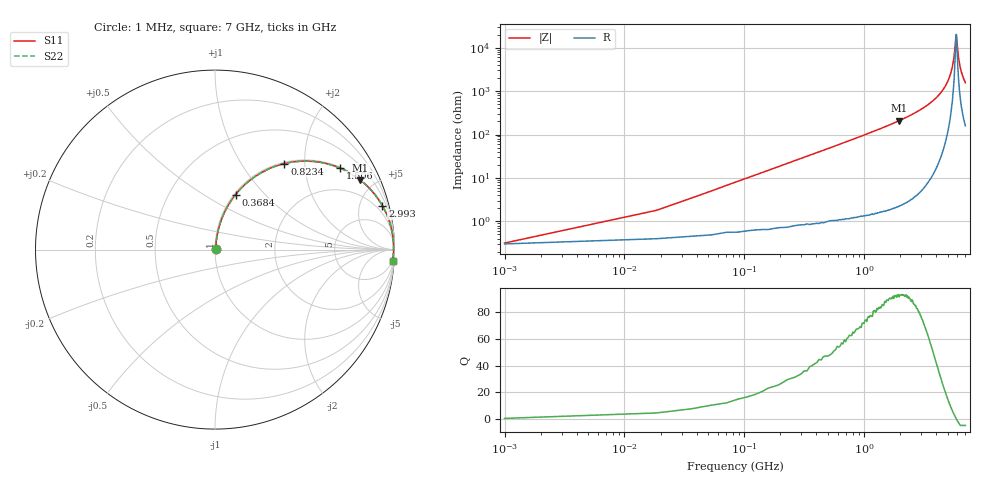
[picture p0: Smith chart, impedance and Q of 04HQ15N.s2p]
! Coilcraft 0403HQ-15N Chip Inductor
! 13 February 2004
# MHZ S MA R 50
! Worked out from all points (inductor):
!   401 points, 1 MHz to 7 GHz, reference 50 ohm
!   read as one part in series: L = 15 nH near 35.99 MHz
!   highest Q = 93 at 1.961 GHz (marker M1), where L = 16.9 nH
!   self-resonance near 5.863 GHz
!   S11 on the Smith chart (normalised r, x): 1 MHz: 1.01, +0.00; 368.4 MHz: 1.02, +0.70; 823.4 MHz: 1.02, +1.58; 1.506 GHz: 1.03, +3.04; 2.993 GHz: 1.10, +7.62; 7 GHz: 4, -31
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1  0.003178 17.1  0.997 -0.1  0.997 -0.1  0.003178 17.1
53.492  0.05 81.4  0.994 -2.9  0.994 -2.9  0.05 81.4
105.985  0.099 80.9  0.989 -5.7  0.989 -5.7  0.099 80.9
210.97  0.194 76.7  0.974 -11.2  0.974 -11.2  0.194 76.7
368.447  0.327 69.5  0.937 -19.1  0.937 -19.1  0.327 69.5
823.382  0.616 51.1  0.778 -38.0  0.778 -38.0  0.616 51.1
1173.332  0.75 40.6  0.651 -48.6  0.651 -48.6  0.75 40.6
1505.785  0.831 33.2  0.547 -56.2  0.547 -56.2  0.831 33.2
1960.72  0.897 25.6  0.431 -63.8  0.431 -63.8  0.897 25.6
2345.665  0.931 20.7  0.354 -68.6  0.354 -68.6  0.931 20.7
2993.072  0.964 14.7  0.253 -74.6  0.253 -74.6  0.964 14.7
3500.5  0.978 11.0  0.191 -78.0  0.191 -78.0  0.978 11.0
4672.833  0.993 4.7  0.083 -82.7  0.083 -82.7  0.993 4.7
5127.768  0.995 2.8  0.049 -82.4  0.049 -82.4  0.995 2.8
5425.225  0.995 1.6  0.029 -79.5  0.029 -79.5  0.995 1.6
5600.2  0.995 1.0  0.018 -73.9  0.018 -73.9  0.995 1.0
5845.165  0.995 0.1  0.005169 -18.5  0.005169 -18.5  0.995 0.1
5897.658  0.995 -0.1  0.005204 17.4  0.005204 17.4  0.995 -0.1
6107.628  0.995 -0.8  0.015 68.9  0.015 68.9  0.995 -0.8
6317.598  0.994 -1.5  0.027 76.7  0.027 76.7  0.994 -1.5
6667.548  0.993 -2.6  0.046 79.9  0.046 79.9  0.993 -2.6
7000  0.992 -3.6  0.064 80.5  0.064 80.5  0.992 -3.6
